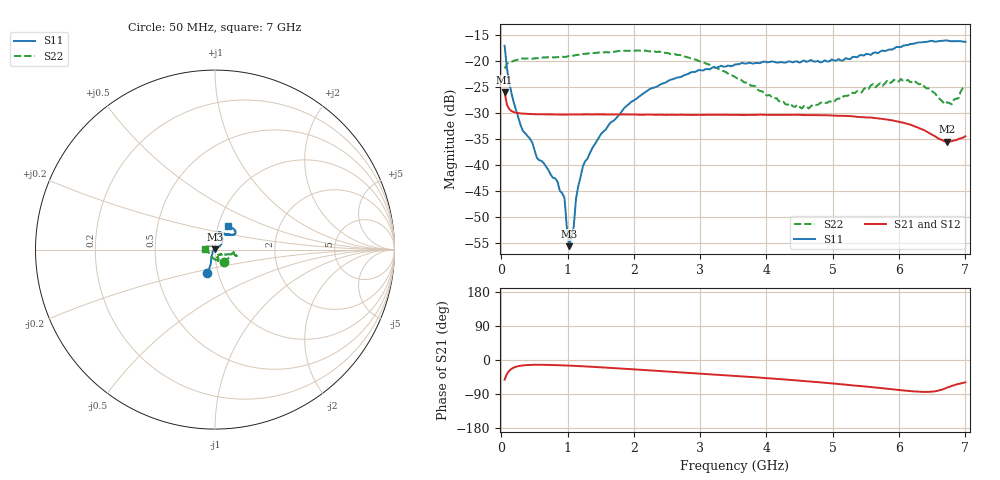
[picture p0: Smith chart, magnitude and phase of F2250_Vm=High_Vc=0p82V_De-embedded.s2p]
! Integrated Device Technology
! Corporate Headquarters
! 6024 Silver Creek Valley Road
! San Jose, CA 95138  USA
! Phone:  1-408-284-8200
! Toll Free:  1-800-223-1366
! Webpage:  http://www.idt.com/
! Timing and RF Division
! 515 Groton Road, Suite 102
! Westford, MA 01886-6024
! Device:  F2250
! Description: Voltage Variable RF Attenuator
! Frequency:  50.0 -  6000.00 MHz
! Package:  3x3 mm Thin QFN Plastic Package: 16 pin
! Ports:  2 RF, 3 DC
!  Pin  1  = GND
!  Pin  2  = NC
!  Pin  3  = RF1  = Port 1
!  Pin  4  = NC
!  Pin  5  = GND
!  Pin  6  = GND
!  Pin  7  = GND
!  Pin  8  = GND
!  Pin  9  = NC
!  Pin 10  = RF2  = Port 2
!  Pin 11  = NC
!  Pin 12  = GND
!  Pin 13  = GND
!  Pin 14  = VCNTRL
!  Pin 15  = VDD
!  Pin 16  = VMODE
! Vcntrl:  0.820 Volts
! Vmode:  +3.300 Volts
! Vdd:  +3.30  Volts
! Current:  1.305 mA
! Data:  The device was measured on a the F2250 evaluation board which has
!  individual transmission lines to the RF pins.  Data was collected
!  using a calibrated network analyzer.  The evaluation board was
!  de-embedded using a TRL calibration technique.
!  The reference plane is the edge of the package pin.
! Misc:  SN 10
!  Action Tracker AT0258
! Date Measured:  2014-11-26
! Date:  2015-10-15  MJV
! Note:
!  Integrated Device Technology supplies this data as a sample of measured
!  data at the package pin for this product.  Your particular data for this
!  product may vary.
!  Data was taken at 25 degrees C.
!  Integrated Device Technology reserves the right to change this data at anytime.
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# GHz S dB R 50
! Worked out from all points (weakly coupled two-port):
!   201 points, 50 MHz to 7 GHz, reference 50 ohm
!   highest |S21| = -26.05 dB at 50 MHz (marker M1); lowest = -35.6 dB at 6.722 GHz (marker M2)
!   lowest |S11| = -55.6 dB at 1.023 GHz (marker M3), VSWR 1.00, Z = 49.9 + j0.137 ohm
!   |S11| at or under -10 dB: start of sweep to end of sweep
!   |S22| runs from -29.2 to -18.1 dB; largest |S21 - S12| = 0.0001
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0.05  -17.15 -107.6  -26.05 -51.9  -26.06 -51.9  -21.53 -55.6
0.1195  -24.21 -110.5  -29.31 -28.3  -29.32 -28.3  -20.37 -16.3
0.29325  -32.47 -124.3  -30.14 -15.1  -30.14 -15.1  -19.63 -9.5
0.467  -35.73 -142.5  -30.27 -12.8  -30.26 -12.8  -19.63 -7.8
0.5365  -38.65 -150.3  -30.30 -12.6  -30.30 -12.6  -19.55 -8.7
0.8145  -42.59 171.3  -30.35 -13.5  -30.36 -13.5  -19.39 -11.5
0.9535  -46.37 173.9  -30.37 -14.3  -30.37 -14.3  -19.32 -13.0
0.98825  -51.99 168.3  -30.35 -14.5  -30.36 -14.6  -19.24 -13.4
1.023  -55.60 123.9  -30.35 -14.8  -30.35 -14.8  -19.12 -13.3
1.0925  -51.88 59.8  -30.35 -15.3  -30.35 -15.3  -19.05 -13.7
1.12725  -46.46 44.5  -30.35 -15.6  -30.34 -15.6  -18.94 -14.3
1.2315  -40.23 33.4  -30.33 -16.5  -30.34 -16.5  -18.74 -15.6
1.6485  -31.87 38.4  -30.35 -20.8  -30.35 -20.8  -18.39 -16.4
2.37825  -24.75 45.3  -30.38 -28.9  -30.39 -28.9  -18.29 -16.4
3.525  -20.74 71.1  -30.43 -42.0  -30.43 -42.0  -23.16 -23.4
4.2895  -20.41 75.3  -30.41 -51.6  -30.42 -51.6  -28.40 -44.6
4.7065  -20.16 71.6  -30.46 -57.5  -30.46 -57.5  -28.42 -62.6
5.85325  -17.85 40.2  -31.39 -76.5  -31.40 -76.6  -24.35 -71.6
6.2355  -16.74 38.7  -32.63 -82.9  -32.62 -83.1  -23.91 -80.3
6.722  -16.14 49.0  -35.55 -72.9  -35.56 -73.0  -27.99 -138.4
6.7915  -16.30 51.0  -35.49 -68.5  -35.48 -68.6  -28.40 -153.4
7  -16.40 62.1  -34.52 -58.9  -34.52 -58.9  -24.93 173.9
